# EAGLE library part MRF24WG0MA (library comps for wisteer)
MRF24WG0MA Wifi module G/B with integrated antenna. http://ww1.microchip.com/downloads/en/DeviceDoc/70686B.pdf
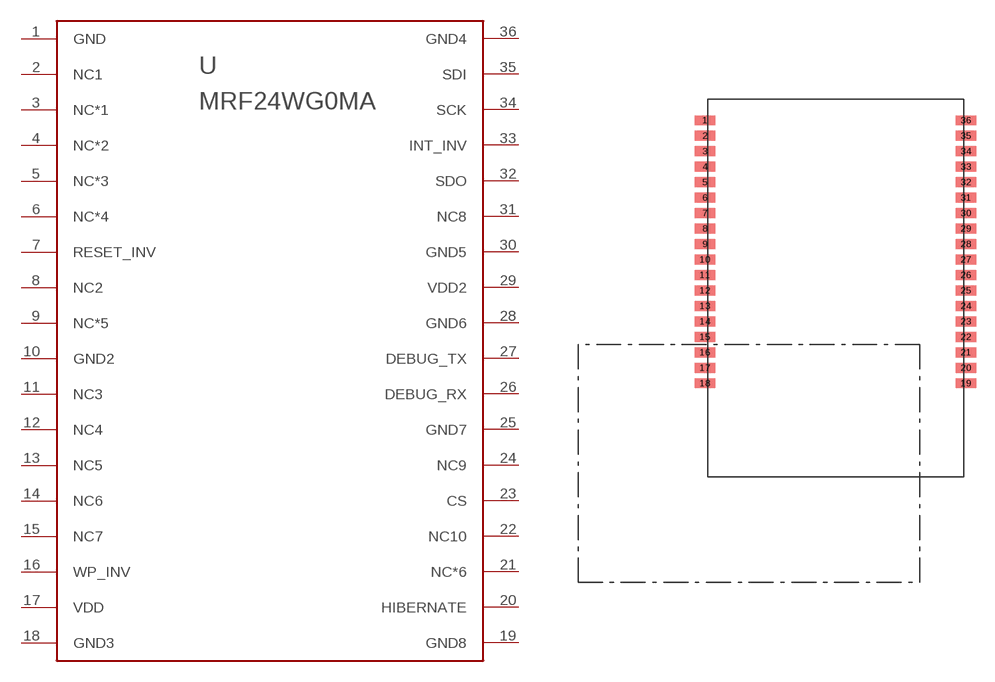
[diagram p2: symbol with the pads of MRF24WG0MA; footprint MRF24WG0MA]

Designator prefix -

## MRF24WG0MA  [MRF24WG0MA]
1  GND  pas
2  NC1  pas
3  NC*1  pas
4  NC*2  pas
5  NC*3  pas
6  NC*4  pas
7  RESET_INV  pas
8  NC2  pas
9  NC*5  pas
10  GND2  pas
11  NC3  pas
12  NC4  pas
13  NC5  pas
14  NC6  pas
15  NC7  pas
16  WP_INV  pas
17  VDD  pas
18  GND3  pas
19  GND8  pas
20  HIBERNATE  pas
21  NC*6  pas
22  NC10  pas
23  CS  pas
24  NC9  pas
25  GND7  pas
26  DEBUG_RX  pas
27  DEBUG_TX  pas
28  GND6  pas
29  VDD2  pas
30  GND5  pas
31  NC8  pas
32  SDO  pas
33  INT_INV  pas
34  SCK  pas
35  SDI  pas
36  GND4  pas

## Footprint MRF24WG0MA (pad centres in mm)
smd 1.7 x 0.8: 1 -10.2,13.27; 2 -10.2,12; 3 -10.2,10.73; 4 -10.2,9.46; 5 -10.2,8.19; 6 -10.2,6.92; 7 -10.2,5.65; 8 -10.2,4.38; 9 -10.2,3.11; 10 -10.2,1.84; 11 -10.2,0.57; 12 -10.2,-0.7; 13 -10.2,-1.97; 14 -10.2,-3.24; 15 -10.2,-4.51; 16 -10.2,-5.78; 17 -10.2,-7.05; 18 -10.2,-8.32; 19 11.2,-8.32; 20 11.2,-7.05; 21 11.2,-5.78; 22 11.2,-4.51; 23 11.2,-3.24; 24 11.2,-1.97; 25 11.2,-0.7; 26 11.2,0.57; 27 11.2,1.84; 28 11.2,3.11; 29 11.2,4.38; 30 11.2,5.65; 31 11.2,6.92; 32 11.2,8.19; 33 11.2,9.46; 34 11.2,10.73; 35 11.2,12; 36 11.2,13.27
